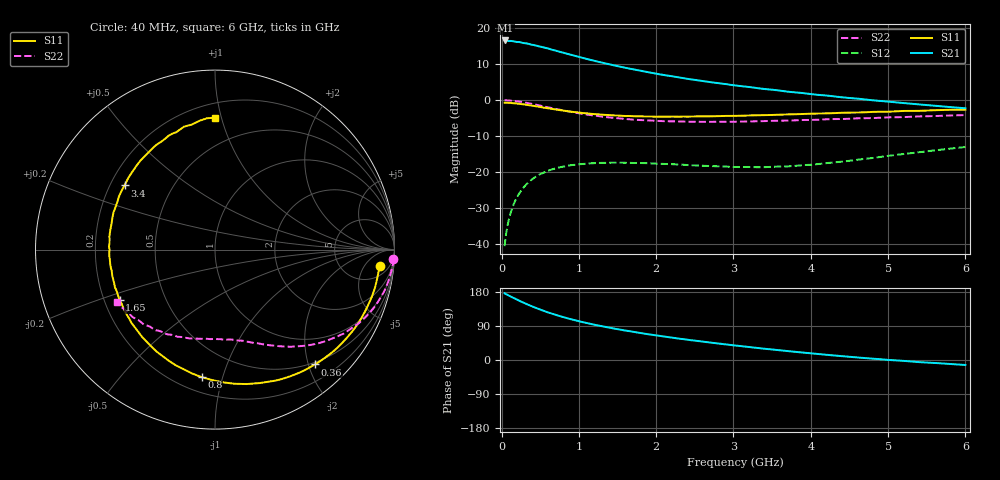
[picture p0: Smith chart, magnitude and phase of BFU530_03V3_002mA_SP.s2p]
! Filename:  P:\Prog\Test\Noise\ATS_data\Testdata_Net\03 Spar\BFU530_APG2013_40_A05_03p3V_002mA_SP_CM01_D.s2p
! Date/Time: Fri 26/Apr/2013 13:03:17
! BFU530_APG2013_40_A05_03p3V_1to25mA_SP_CM01_Bias2_R.s2p
! MDIF S-parameter v. bias file
! BFU530_APG2013_40_A05_03p3V_1to25mA_SP_CM01
! Date/time Wed Apr 24 18:17:07 2013
! VAR V_out= 3.3000
! VAR I_out= 2.0000
! VAR V_in= 0.8003
! VAR I_in= 0.0217
! Device data file deembeded for feedlines and parallel
! Original file: \03 Spar\BFU530_APG2013_40_A05_03p3V_002mA_SP_CM01_R.s2p
! Feed-files: PR047V01_250413_Feed1.s2p, PR047V01_250413_Feed2.s2p
! Parallel-file: PR047V01_250413_Par.s2p
# MHz S MA R 50
!  Freq-MHz  S11-mag  S11-arg  S21-mag  S21-arg  S12-mag  S12-arg  S22-mag  S22-arg
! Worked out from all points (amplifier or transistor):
!   98 points, 40 MHz to 6 GHz, reference 50 ohm
!   highest |S21| = 16.6 dB at 50 MHz (marker M1)
!   |S21| within 3 dB of that: start of sweep to 727.4 MHz
!   unconditionally stable (mu >= 1): 2.87 GHz to 4.921 GHz
!   at 300 MHz: K = 0.11, MSG = 19.9 dB, |S12| = -23.9 dB
!   at 1.6 GHz: K = 0.55, MSG = 13.2 dB, |S12| = -17.4 dB
!   at 6 GHz: K = 0.84, MSG = 5.4 dB, |S12| = -13.0 dB
!   S11 on the Smith chart (normalised r, x): 40 MHz: 10, -12; 360 MHz: 0.46, -2.11; 800 MHz: 0.29, -0.86; 1.65 GHz: 0.26, -0.23; 3.4 GHz: 0.26, +0.30; 6 GHz: 0.30, +0.96
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40  0.9222 -5.7  6.744 176.0  0.009293 86.1  0.9957 -3.0
50  0.92 -7.1  6.754 174.3  0.01161 85.7  0.9972 -3.8
90  0.9163 -12.7  6.626 170.4  0.02069 82.2  0.9895 -7.1
120  0.9121 -17.0  6.659 167.3  0.02743 79.6  0.9837 -9.6
240  0.8845 -33.5  6.39 155.4  0.05247 69.8  0.9492 -18.8
360  0.8481 -49.0  6.021 144.6  0.07366 61.0  0.901 -27.0
440  0.8227 -58.7  5.757 137.8  0.08551 55.7  0.8651 -31.8
550  0.7843 -71.5  5.388 129.3  0.09852 49.1  0.8142 -37.8
700  0.7405 -86.8  4.879 119.2  0.1121 41.6  0.7537 -44.7
800  0.7145 -96.0  4.559 113.1  0.1189 37.6  0.7168 -48.6
900  0.689 -104.6  4.266 107.5  0.1244 33.9  0.6865 -52.1
1050  0.661 -116.3  3.868 99.9  0.1292 29.0  0.6419 -56.9
1200  0.6385 -126.8  3.523 93.1  0.1326 25.1  0.6084 -60.9
1350  0.6221 -136.0  3.227 87.1  0.1342 21.9  0.5807 -64.5
1650  0.6012 -152.2  2.749 76.2  0.1341 17.0  0.5415 -71.1
2050  0.589 -170.2  2.279 63.5  0.1299 13.3  0.5113 -79.0
2500  0.5929 173.0  1.912 51.1  0.1237 12.3  0.4996 -87.4
3100  0.6059 153.6  1.563 36.5  0.1171 16.4  0.5028 -98.5
3400  0.6179 144.7  1.426 29.7  0.1165 19.8  0.5102 -104.2
4100  0.6503 127.5  1.181 15.8  0.129 29.1  0.533 -117.1
5200  0.7065 104.2  0.9097 -2.3  0.1778 34.5  0.58 -137.4
6000  0.7346 89.9  0.7696 -13.2  0.2227 31.3  0.619 -151.9
